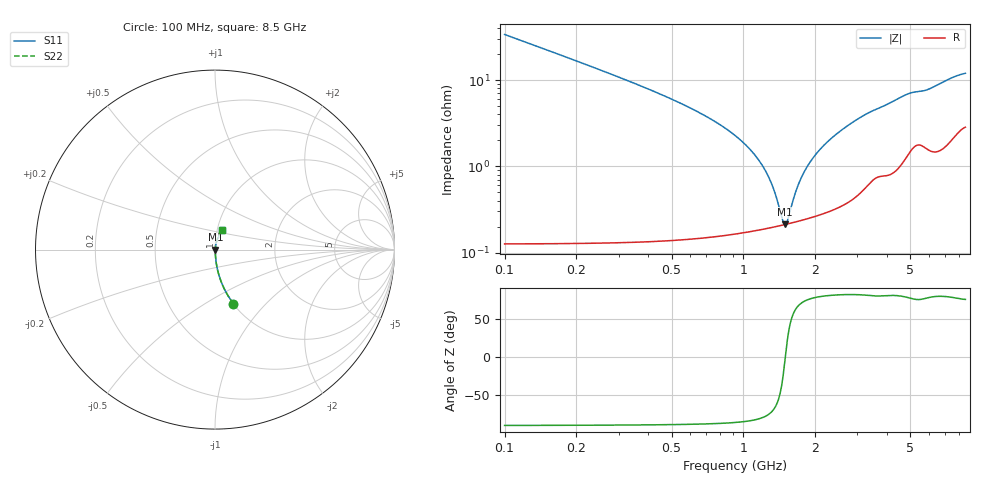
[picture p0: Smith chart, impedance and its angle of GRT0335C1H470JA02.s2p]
!Murata Part Number: GRT0335C1H470JA02
!These Parameters are Measured in Series Mode Connection
!Data Generated on Jun 19, 2026
!  o--ll--o
!Port1  Port2
!  o------o
!Operation Temp=25[degC], DC Bias Voltage=0[V]
!Freq. Start=100[MHz] Stop=9[GHz] 401[Steps]
# Hz S RI R 50
!Freq.(Hz) S11(Real) S11(Imag) S21(Real) S21(Imag) S12(Real) S12(Imag) S22(Real) S22(Imag)
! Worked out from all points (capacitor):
!   401 points, 100 MHz to 8.5 GHz, reference 50 ohm
!   read as one part in series: C = 47 pF near 142 MHz
!   lowest |Z| = 214 mohm at 1.486 GHz (marker M1)
!   series resonance near 1.497 GHz, so ESL is about 240 pH
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1e8  0.1029 -0.302  0.8971 0.302  0.8971 0.302  0.1029 -0.302
2.26e8  0.0222 -0.143  0.9778 0.143  0.9778 0.143  0.0222 -0.143
3.73e8  0.00849 -0.0843  0.9915 0.0843  0.9915 0.0843  0.00849 -0.0843
9.82e8  0.00206 -0.0195  0.9979 0.0195  0.9979 0.0195  0.00206 -0.0195
1.171e9  0.00196 -0.0112  0.998 0.0112  0.998 0.0112  0.00196 -0.0112
1.297e9  0.00198 -0.00647  0.998 0.00647  0.998 0.00647  0.00198 -0.00647
1.444e9  0.00207 -0.00163  0.9979 0.00163  0.9979 0.00163  0.00207 -0.00163
1.486e9  0.00211 -0.000337  0.9979 0.000337  0.9979 0.000337  0.00211 -0.000337
1.507e9  0.00212 0.000293  0.9979 -0.000293  0.9979 -0.000293  0.00212 0.000293
1.549e9  0.00217 0.00153  0.9978 -0.00153  0.9978 -0.00153  0.00217 0.00153
1.633e9  0.00226 0.00391  0.9977 -0.00391  0.9977 -0.00391  0.00226 0.00391
1.717e9  0.00236 0.00618  0.9976 -0.00618  0.9976 -0.00618  0.00236 0.00618
1.822e9  0.00251 0.00889  0.9975 -0.00889  0.9975 -0.00889  0.00251 0.00889
1.969e9  0.00275 0.0125  0.9973 -0.0125  0.9973 -0.0125  0.00275 0.0125
2.347e9  0.00351 0.021  0.9965 -0.021  0.9965 -0.021  0.00351 0.021
2.914e9  0.00533 0.0328  0.9947 -0.0328  0.9947 -0.0328  0.00533 0.0328
3.376e9  0.00802 0.0413  0.992 -0.0413  0.992 -0.0413  0.00802 0.0413
4.3e9  0.0118 0.0563  0.9882 -0.0563  0.9882 -0.0563  0.0118 0.0563
4.951e9  0.0186 0.0663  0.9814 -0.0663  0.9814 -0.0663  0.0186 0.0663
5.707e9  0.0215 0.0706  0.9785 -0.0706  0.9785 -0.0706  0.0215 0.0706
7.114e9  0.0263 0.0941  0.9737 -0.0941  0.9737 -0.0941  0.0263 0.0941
8.5e9  0.0399 0.1085  0.9601 -0.1085  0.9601 -0.1085  0.0399 0.1085
